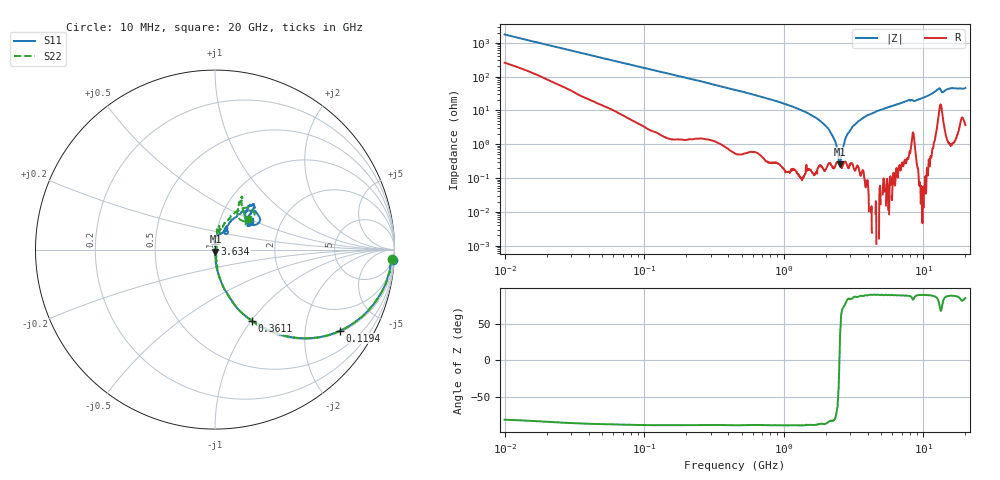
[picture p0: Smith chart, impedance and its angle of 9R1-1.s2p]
!Keysight Technologies,P5008B,MY61100088,A.16.20.02
!Date: Monday, May 27, 2024 16:57:09
!Correction: S11(C* 2-Port  )
!S21(C* 2-Port  )
!S12(C* 2-Port  )
!S22(C* 2-Port  )
!S2P File: Measurements: S11, S21, S12, S22:Log Frequency Sweep
# Hz S  dB  R 50
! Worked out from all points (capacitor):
!   1601 points, 10 MHz to 20 GHz, reference 50 ohm
!   read as one part in series: C = 9.15 pF near 10.39 MHz
!   lowest |Z| = 258 mohm at 2.509 GHz (marker M1)
!   series resonance near 2.504 GHz, so ESL is about 440 pH
!   S11 on the Smith chart (normalised r, x): 10 MHz: 5, -35; 119.4 MHz: 1.05, -3.05; 361.1 MHz: 1.02, -1.01; 3.634 GHz: 1.00, +0.06; 20 GHz: 1.38, +0.48
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1e7  -0.07 -3.2  -25.01 78.4  -25.02 78.4  -0.09 -3.2
3.555162e7  -0.26 -11.2  -14.13 75.7  -14.14 75.7  -0.27 -11.3
1.193881e8  -1.61 -33.0  -5.30 56.2  -5.31 56.2  -1.61 -33.0
1.263918e8  -1.76 -34.4  -4.97 54.8  -4.99 54.8  -1.75 -34.5
2.071504e8  -3.57 -47.8  -2.63 41.4  -2.65 41.4  -3.58 -47.7
3.611383e8  -6.99 -62.5  -1.05 26.4  -1.06 26.4  -6.99 -62.6
4.472136e8  -8.52 -67.5  -0.71 21.8  -0.72 21.8  -8.51 -67.6
9.076605e8  -14.73 -79.2  -0.17 10.0  -0.18 10.0  -14.75 -79.0
1.589917e9  -22.31 -85.9  -0.03 3.6  -0.04 3.6  -22.15 -83.4
2.054869e9  -27.74 -86.2  -0.01 1.2  -0.02 1.1  -27.33 -80.1
2.347211e9  -32.41 -84.7  0.00 -0.1  -0.01 -0.1  -31.77 -74.6
2.508627e9  -38.27 -77.1  0.00 -0.8  -0.01 -0.8  -36.40 -63.6
2.838428e9  -48.59 52.4  0.00 -2.0  -0.01 -2.0  -42.18 23.4
3.136201e9  -36.20 81.9  0.00 -3.0  -0.01 -3.0  -34.21 63.1
3.633803e9  -29.98 89.6  0.00 -4.5  -0.01 -4.6  -28.28 71.6
5.652411e9  -21.88 78.5  -0.01 -9.8  -0.02 -9.8  -21.95 80.4
7.697294e9  -17.73 61.8  -0.06 -15.0  -0.07 -15.1  -17.96 80.9
9.264046e9  -18.94 62.9  -0.03 -17.9  -0.04 -18.0  -18.86 77.3
1.27966e10  -10.36 45.2  -0.83 -29.7  -0.84 -29.6  -10.55 52.2
1.380717e10  -12.36 45.2  -0.65 -24.5  -0.66 -24.6  -12.79 55.6
1.592205e10  -9.62 49.1  -0.50 -31.9  -0.51 -31.9  -9.75 61.9
2e10  -12.00 40.1  -0.53 -39.2  -0.54 -39.2  -11.94 43.1
